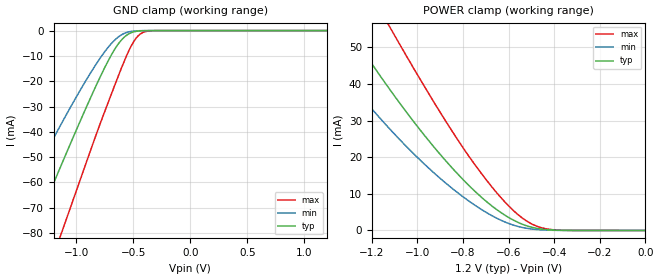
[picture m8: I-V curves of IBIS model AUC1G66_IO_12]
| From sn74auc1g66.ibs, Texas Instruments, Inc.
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[Model]   AUC1G66_IO_12
Model_type  Terminator
| variable   typ   min   max
C_comp   2.99pF   2.71pF   3.14pF
| C_tri-state   2.99pF   2.71pF   3.14pF
[Temperature Range]   40   100   -40
| Ambient temperature   25   85   -40
[Voltage range]   1.2   1.1   1.3
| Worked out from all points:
|   GND clamp passes 1 mA (typ) near -0.53 V on its own axis
|   POWER clamp passes 1 mA (typ) near -0.51 V on its own axis
[GND Clamp]
| AUC1G66_IO_12
|   Voltage   I(typ)   I(min)   I(max)
-2.7V     -221.8mA   -178.5mA   -275mA
-1.645V   -108.3mA   -81.52mA   -144.9mA
-1.6V     -103.4mA   -77.48mA   -139.3mA
-1.4V     -81.83mA   -59.74mA   -114.2mA
-1.36V    -77.52mA   -56.25mA   -109.1mA
-1.13V    -52.92mA   -36.7mA    -79.94mA
-785mV    -17.79mA   -10.5mA    -36.08mA
-670mV    -7.884mA   -4.059mA   -22.43mA
-580mV    -2.621mA   -1.126mA   -12.14mA
-475mV    -310.4uA   -114.6uA   -2.98mA
-370mV    -17.52uA   -7.845uA   -194uA
1.2V      283.4pA    8.137nA    163.3pA
[POWER Clamp]
| AUC1G66_IO_12
|   Voltage   I(typ)   I(min)   I(max)
-2.7V     211.1mA    181.9mA    241.3mA
-1.48V    72.52mA    55.24mA    96.17mA
-1.31V    55.75mA    41.41mA    76.64mA
-1.285V   53.38mA    39.49mA    73.8mA
-1.125V   38.83mA    27.95mA    55.96mA
-1.105V   37.1mA     26.61mA    53.78mA
-940mV    23.72mA    16.42mA    36.29mA
-795mV    13.58mA    8.96mA     22.12mA
-650mV    5.596mA    3.28mA     10.13mA
-545mV    1.833mA    886.2uA    3.634mA
-420mV    160.1uA    72.28uA    303uA
-35.59fV  283.4pA    564.1pA    190.3pA
